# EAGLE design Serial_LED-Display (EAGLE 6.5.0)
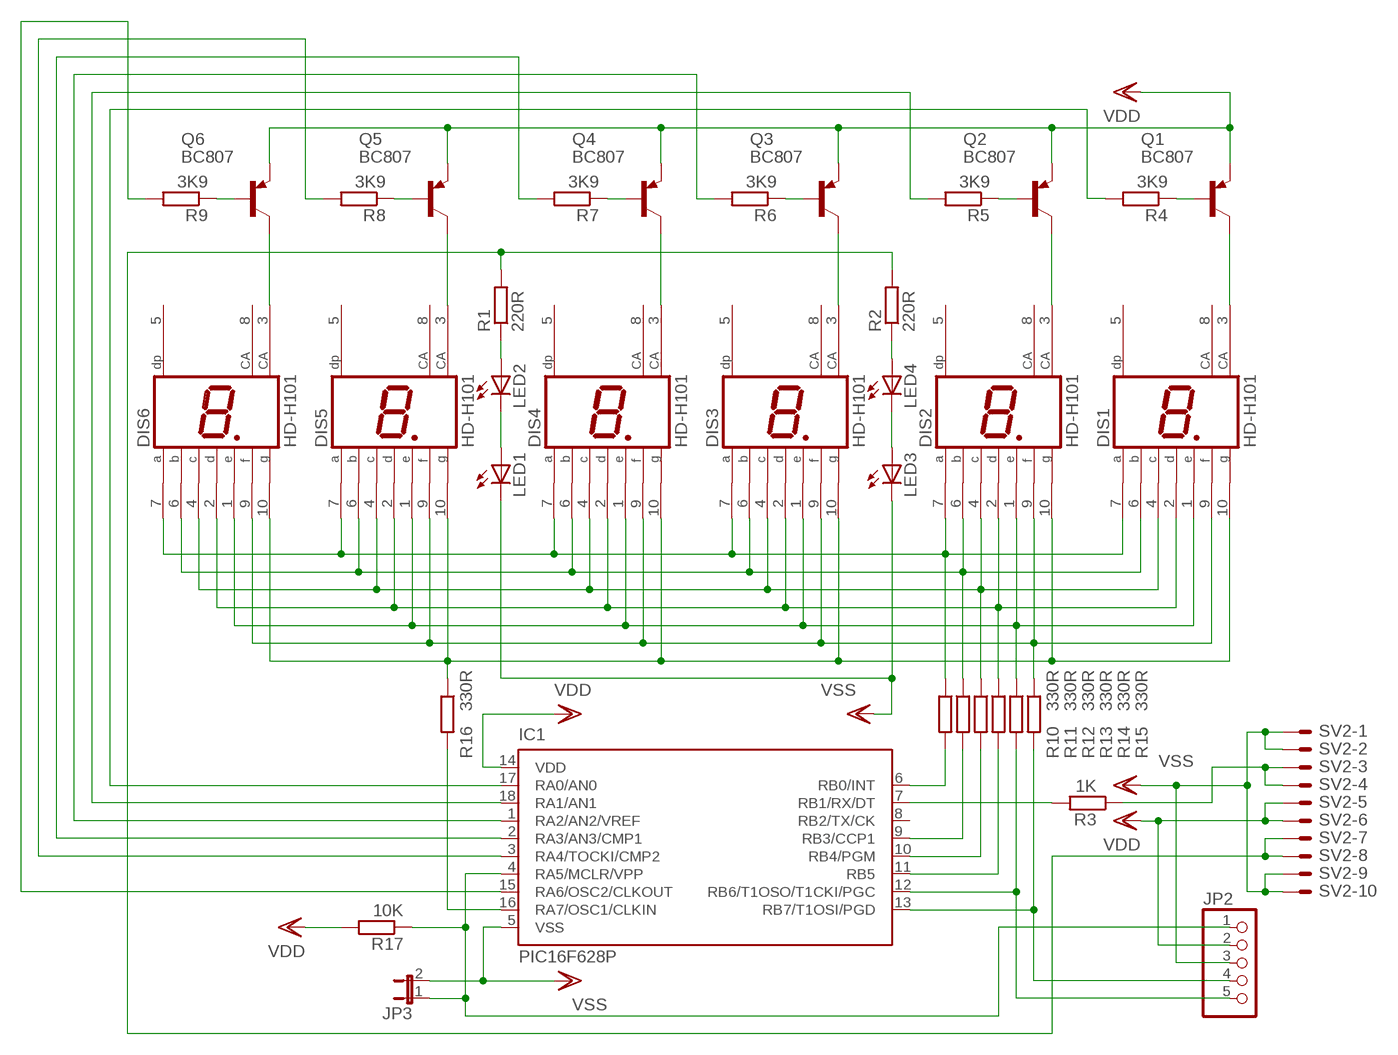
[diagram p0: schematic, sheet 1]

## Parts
DIS1  HD-H101  [HDSP-M]
DIS2  HD-H101  [HDSP-M]
DIS3  HD-H101  [HDSP-M]
DIS4  HD-H101  [HDSP-M]
DIS5  HD-H101  [HDSP-M]
DIS6  HD-H101  [HDSP-M]
IC1  PIC16F628P  [DIL18]
JP2  PINHD-1X5  [1X05]
JP3  JP1E  [JP1]
LED1  LED3MM  [LED3MM]
LED2  LED3MM  [LED3MM]
LED3  LED3MM  [LED3MM]
LED4  LED3MM  [LED3MM]
Q1  BC807  BC807-25SMD  [SOT23-BEC]
Q2  BC807  BC807-25SMD  [SOT23-BEC]
Q3  BC807  BC807-25SMD  [SOT23-BEC]
Q4  BC807  BC807-25SMD  [SOT23-BEC]
Q5  BC807  BC807-25SMD  [SOT23-BEC]
Q6  BC807  BC807-25SMD  [SOT23-BEC]
R1  220R  R-EU_R1206  [R1206]
R2  220R  R-EU_R1206  [R1206]
R3  1K  R-EU_R1206  [R1206]
R4  3K9  R-EU_R1206  [R1206]
R5  3K9  R-EU_R1206  [R1206]
R6  3K9  R-EU_R1206  [R1206]
R7  3K9  R-EU_R1206  [R1206]
R8  3K9  R-EU_R1206  [R1206]
R9  3K9  R-EU_R1206  [R1206]
R10  330R  R-EU_R1206  [R1206]
R11  330R  R-EU_R1206  [R1206]
R12  330R  R-EU_R1206  [R1206]
R13  330R  R-EU_R1206  [R1206]
R14  330R  R-EU_R1206  [R1206]
R15  330R  R-EU_R1206  [R1206]
R16  330R  R-EU_R1206  [R1206]
R17  10K  R-EU_R1206  [R1206]
SV2  ML10E  [ML10]

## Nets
N$1: DIS1.7(A) DIS2.7(A) DIS3.7(A) DIS4.7(A) DIS5.7(A) DIS6.7(A) R10.1
N$2: DIS1.6(B) DIS2.6(B) DIS3.6(B) DIS4.6(B) DIS5.6(B) DIS6.6(B) R11.1
N$3: DIS1.4(C) DIS2.4(C) DIS3.4(C) DIS4.4(C) DIS5.4(C) DIS6.4(C) R12.1
N$4: DIS1.2(D) DIS2.2(D) DIS3.2(D) DIS4.2(D) DIS5.2(D) DIS6.2(D) R13.1
N$5: DIS1.1(E) DIS2.1(E) DIS3.1(E) DIS4.1(E) DIS5.1(E) DIS6.1(E) R14.1
N$6: DIS1.9(F) DIS2.9(F) DIS3.9(F) DIS4.9(F) DIS5.9(F) DIS6.9(F) R15.1
N$7: DIS1.10(G) DIS2.10(G) DIS3.10(G) DIS4.10(G) DIS5.10(G) DIS6.10(G) R16.1
N$8: IC1.4(RA5/MCLR/VPP) JP2.1 JP3.1 R17.1
N$9: LED1.A LED2.K(C)
N$10: LED3.A LED4.K(C)
N$11: LED2.A R1.1
N$12: LED4.A R2.1
N$15: DIS1.3(CA) Q1.C
N$16: DIS2.3(CA) Q2.C
N$17: DIS3.3(CA) Q3.C
N$18: IC1.7(RB1/RX/DT) R3.2
N$19: DIS4.3(CA) Q4.C
N$20: DIS5.3(CA) Q5.C
N$21: DIS6.3(CA) Q6.C
N$22: Q6.B R9.1
N$23: Q5.B R8.1
N$24: Q4.B R7.1
N$25: Q3.B R6.1
N$26: Q2.B R5.1
N$27: Q1.B R4.1
N$28: IC1.17(RA0/AN0) R4.2
N$29: IC1.18(RA1/AN1) R5.2
N$30: IC1.1(RA2/AN2/VREF) R6.2
N$31: IC1.2(RA3/AN3/CMP1) R7.2
N$32: IC1.3(RA4/TOCKI/CMP2) R8.2
N$33: IC1.15(RA6/OSC2/CLKOUT) R9.2
N$34: IC1.9(RB3/CCP1) R11.2
N$35: IC1.6(RB0/INT) R10.2
N$36: IC1.10(RB4/PGM) R12.2
N$37: IC1.11(RB5) R13.2
N$38: IC1.12(RB6/T1OSO/T1CKI/PGC) JP2.5 R14.2
N$39: IC1.13(RB7/T1OSI/PGD) JP2.4 R15.2
N$40: IC1.16(RA7/OSC1/CLKIN) R16.2
N$45: R3.1 SV2.3 SV2.4
N$47: R1.2 R2.2 SV2.7 SV2.8
VDD: IC1.14(VDD) JP2.2 Q1.E Q2.E Q3.E Q4.E Q5.E Q6.E R17.2 SV2.5 SV2.6
VSS: IC1.5(VSS) JP2.3 JP3.2 LED1.K(C) LED3.K(C) SV2.1 SV2.2 SV2.9 SV2.10
Unconnected: DIS1.5(DP) DIS1.8(CA) DIS2.5(DP) DIS2.8(CA) DIS3.5(DP) DIS3.8(CA) DIS4.5(DP) DIS4.8(CA) DIS5.5(DP) DIS5.8(CA) DIS6.5(DP) DIS6.8(CA) IC1.8(RB2/TX/CK)

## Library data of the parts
DIS1-DIS6 = display-hp:HD-H101: LED DISPLAY 1-character 7 segment, decimal point right; OC_FARNELL: unknown; OC_NEWARK: unknown
IC1 = microchip-6:PIC16F62*: FLASH-Based 8-Bit CMOS Microcontroller Source: http://ww1.microchip.com/downloads/en/DeviceDoc/40300C.pdf
JP2 = pinhead:PINHD-1X5: PIN HEADER
JP3 = jumper:JP1E: JUMPER
LED1-LED4 = led:LED: LED
Q1-Q6 = transistor-pnp:BC807*: PNP Transistror
R1-R17 = rcl:R-EU_: RESISTOR, European symbol
SV2 = con-ml:ML10E: HARTING; OC_FARNELL: unknown; OC_NEWARK: unknown

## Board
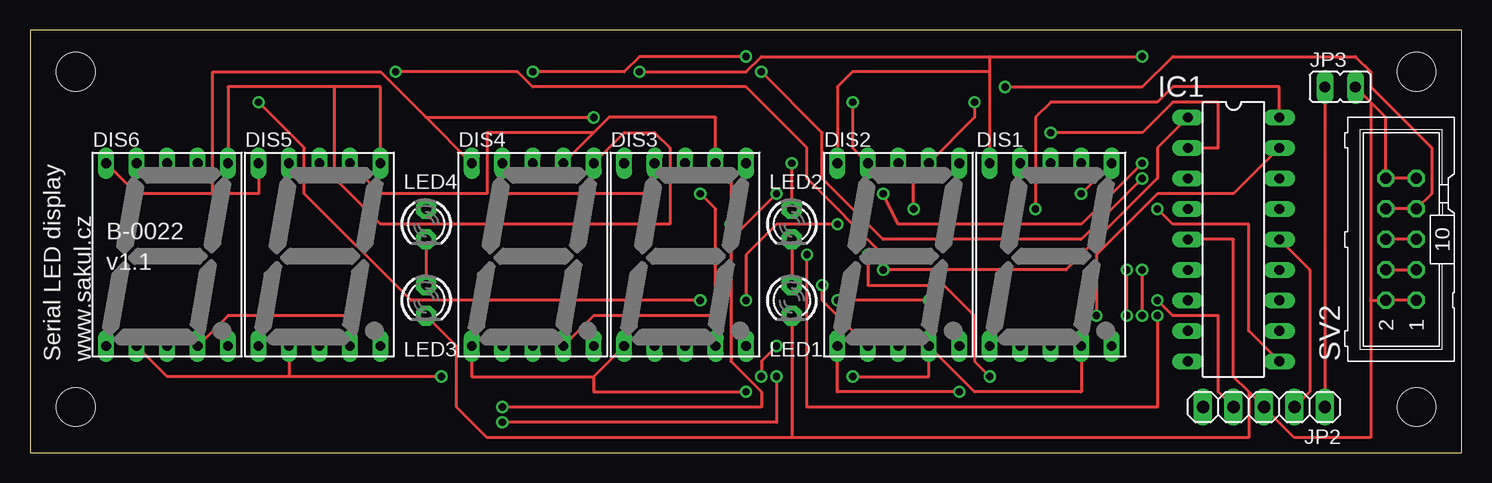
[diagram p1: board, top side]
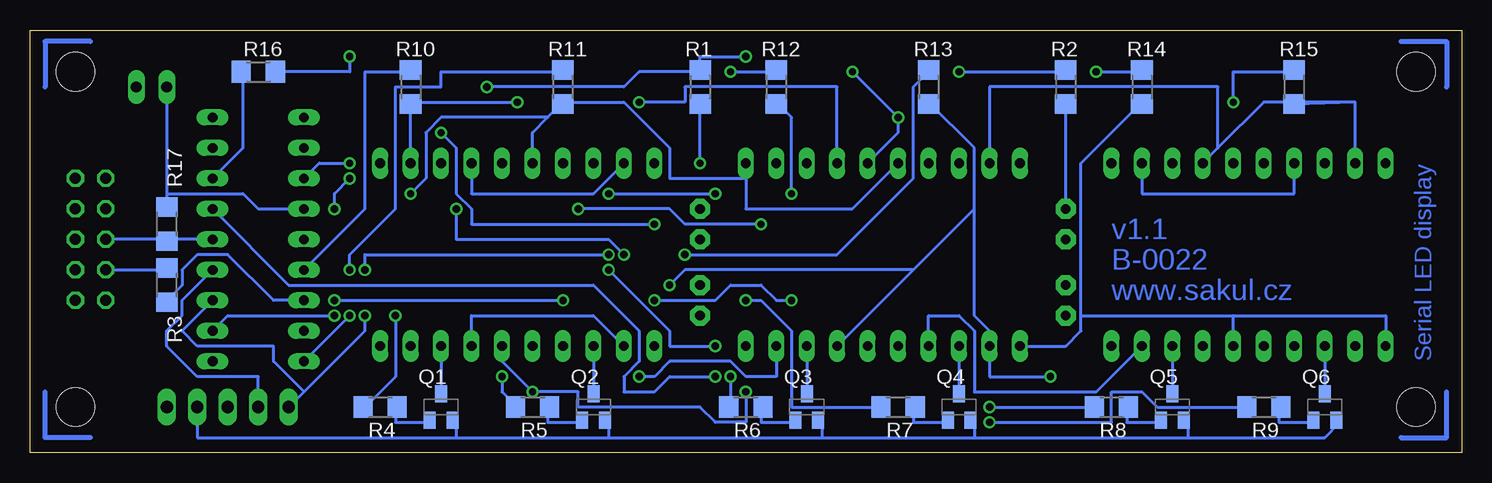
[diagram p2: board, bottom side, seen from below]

Size 119.36 x 35.23 mm. Coordinates in mm from the lower left corner, seen from the top.
Outline: 0,0 119.36,0 119.36,35.23 0,35.23 0,0
Copper layers (1*16): Top 0.035mm / dielectric 1.5mm / Bottom 0.035mm
Design rules "default": minimum track width 10mil, minimum drill 24mil, track to track 8mil, track to pad 8mil, pad to pad 8mil, via to via 8mil, smd to smd 8mil, copper to edge 40mil, drill to drill 8mil, minimum pad ring 10mil, minimum via ring 8mil, stop-mask expansion 4mil, vias tented up to drill 0mil, thermal gap 10mil
Holes 3.2 mm at 3.81,31.75 3.81,3.81 115.57,31.75 115.57,3.81

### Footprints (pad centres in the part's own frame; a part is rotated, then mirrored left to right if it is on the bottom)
HDSP-M = drill 0.813 long: 1 -5.08,-7.62; 2 -2.54,-7.62; 3 0,-7.62; 4 2.54,-7.62; 5 5.08,-7.62; 6 5.08,7.62; 7 2.54,7.62; 8 0,7.62; 9 -2.54,7.62; 10 -5.08,7.62
DIL18 = drill 0.813 long: 1 -10.16,-3.81; 2 -7.62,-3.81; 3 -5.08,-3.81; 4 -2.54,-3.81; 5 0,-3.81; 6 2.54,-3.81; 7 5.08,-3.81; 8 7.62,-3.81; 9 10.16,-3.81; 10 10.16,3.81; 11 7.62,3.81; 12 5.08,3.81; 13 2.54,3.81; 14 0,3.81; 15 -2.54,3.81; 16 -5.08,3.81; 17 -7.62,3.81; 18 -10.16,3.81
1X05 = drill 1.016 long: 1 -5.08,0; 2 -2.54,0; 3 0,0; 4 2.54,0; 5 5.08,0
JP1 = drill 0.914 long: 1 0,-1.27; 2 0,1.27
LED3MM = drill 0.813 pad 1.676 octagon: A -1.27,0; K 1.27,0
SOT23-BEC = smd 1 x 1.4: B -0.95,-1.1; C 0,1.1; E 0.95,-1.1
R1206 = smd 1.6 x 1.803: 1 -1.422,0; 2 1.422,0
ML10 = drill 0.914 octagon: 1 -5.08,-1.27; 2 -5.08,1.27; 3 -2.54,-1.27; 4 -2.54,1.27; 5 0,-1.27; 6 0,1.27; 7 2.54,-1.27; 8 2.54,1.27; 9 5.08,-1.27; 10 5.08,1.27

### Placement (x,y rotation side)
DIS1  85.09,16.51 0 top
DIS2  72.39,16.51 0 top
DIS3  54.61,16.51 0 top
DIS4  41.91,16.51 0 top
DIS5  24.13,16.51 0 top
DIS6  11.43,16.51 0 top
IC1  100.33,17.78 270 top
JP2  102.87,3.81 180 top
JP3  109.22,30.48 270 top
LED1  63.5,12.7 270 top
LED2  63.5,19.05 270 top
LED3  33.02,12.7 270 top
LED4  33.02,19.05 270 top
Q1  85.09,3.81 0 bottom
Q2  72.39,3.81 0 bottom
Q3  54.61,3.81 0 bottom
Q4  41.91,3.81 0 bottom
Q5  24.13,3.81 0 bottom
Q6  11.43,3.81 0 bottom
R1  63.5,30.48 90 bottom
R2  33.02,30.48 90 bottom
R3  107.95,13.97 270 bottom
R4  90.17,3.81 180 bottom
R5  77.47,3.81 180 bottom
R6  59.69,3.81 180 bottom
R7  46.99,3.81 180 bottom
R8  29.21,3.81 180 bottom
R9  16.51,3.81 180 bottom
R10  87.63,30.48 90 bottom
R11  74.93,30.48 90 bottom
R12  57.15,30.48 90 bottom
R13  44.45,30.48 90 bottom
R14  26.67,30.48 90 bottom
R15  13.97,30.48 90 bottom
R16  100.33,31.75 180 bottom
R17  107.95,19.05 270 bottom
SV2  114.3,17.78 90 top

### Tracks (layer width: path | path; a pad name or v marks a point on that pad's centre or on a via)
N$1  (via drill 0.61)
  Top 0.254: v78.74,29.21 78.74,27.94 DIS2.7 73.66,22.86 v73.66,20.32 | 46.99,26.67 48.26,27.94 57.15,27.94 DIS3.7 58.42,22.86 v58.42,19.05 | 46.99,26.67 DIS4.7 | DIS5.7 29.21,21.59 38.1,21.59 38.1,26.67 46.99,26.67
  Bottom 0.254: DIS1.7 R10.1 87.63,29.21 v78.74,29.21 | DIS6.7 13.97,21.59 26.67,21.59 DIS5.7 | v73.66,20.32 66.04,20.32 64.77,19.05 v58.42,19.05
N$2  (via drill 0.61)
  Top 0.254: DIS6.6 16.51,30.48 25.4,30.48 | 25.4,30.48 29.21,30.48 DIS5.6 | v87.63,21.59 DIS1.6 | 25.4,30.48 25.4,22.86 29.21,19.05 53.34,19.05 53.34,25.4 52.07,26.67 49.53,26.67 DIS4.6
  Bottom 0.254: DIS4.6 50.8,20.32 59.69,20.32 59.69,22.86 | 76.2,27.94 77.47,26.67 DIS2.6 | 76.2,27.94 74.93,29.21 | v87.63,21.59 86.36,22.86 86.36,26.67 85.09,27.94 76.2,27.94 | 59.69,22.86 66.04,22.86 66.04,25.4 69.85,29.21 74.93,29.21 | 59.69,22.86 DIS3.6 | 74.93,29.21 R11.1
N$3  (via drill 0.61)
  Top 0.254: DIS1.4 87.63,5.08 78.74,5.08 DIS2.4 74.93,6.35 v68.58,6.35 | DIS6.4 16.51,11.43 26.67,11.43 DIS5.4 | v55.88,21.59 57.15,20.32 57.15,11.43 | DIS3.4 57.15,11.43 | DIS4.4 46.99,11.43 57.15,11.43
  Bottom 0.254: v55.88,21.59 55.88,27.94 57.15,29.21 R12.1 | DIS5.4 30.48,5.08 40.64,5.08 40.64,10.16 41.91,11.43 44.45,11.43 DIS4.4 | v68.58,6.35 67.31,6.35 66.04,7.62 60.96,7.62 59.69,6.35 57.15,6.35 DIS3.4
N$4  (via drill 0.61)
  Top 0.254: DIS6.2 11.43,6.35 21.59,6.35 | DIS5.2 21.59,6.35 | v34.29,6.35 21.59,6.35 | DIS2.2 66.04,12.7 v66.04,13.97
  Bottom 0.254: DIS2.2 72.39,11.43 82.55,11.43 DIS1.2 | 40.64,20.32 40.64,11.43 39.37,10.16 DIS4.2 39.37,6.35 v34.29,6.35 | 40.64,20.32 40.64,25.4 44.45,29.21 R13.1 | 40.64,20.32 45.72,15.24 | 45.72,15.24 DIS3.2 | v66.04,13.97 64.77,15.24 45.72,15.24
N$5  (via drill 0.61)
  Top 0.254: DIS2.1 67.31,5.08 v77.47,5.08 | 46.99,6.35 DIS3.1 | 46.99,6.35 36.83,6.35 DIS4.1 | v59.69,5.08 46.99,5.08 46.99,6.35
  Bottom 0.254: DIS1.1 80.01,7.62 v77.47,5.08 73.66,5.08 73.66,3.81 63.5,3.81 62.23,2.54 59.69,2.54 v59.69,5.08 | DIS6.1 6.35,11.43 19.05,11.43 | DIS5.1 19.05,11.43 | 31.75,11.43 31.75,10.16 33.02,8.89 DIS4.1 | 31.75,11.43 31.75,24.13 26.67,29.21 R14.1 | 31.75,11.43 19.05,11.43
N$6  (via drill 0.61)
  Top 0.254: DIS4.9 39.37,21.59 52.07,21.59 DIS3.9 | DIS2.9 68.58,25.4 v68.58,29.21
  Bottom 0.254: DIS2.9 72.39,21.59 82.55,21.59 DIS1.9 | DIS6.9 8.89,29.21 | 20.32,25.4 16.51,29.21 8.89,29.21 | 20.32,25.4 DIS5.9 | 8.89,29.21 R15.1 | DIS4.9 39.37,30.48 20.32,30.48 20.32,25.4 | v68.58,29.21 64.77,29.21 64.77,30.48 52.07,30.48 DIS3.9
N$7  (via drill 0.61)
  Top 0.254: 80.01,33.02 v92.71,33.02 | DIS1.10 80.01,31.75 | 80.01,31.75 80.01,33.02 | DIS2.10 67.31,30.48 68.58,31.75 80.01,31.75 | DIS6.10 8.89,21.59 15.24,21.59 | 15.24,21.59 19.05,21.59 DIS5.10 | 33.02,27.94 29.21,31.75 15.24,31.75 15.24,21.59 | 33.02,27.94 DIS4.10 | 33.02,27.94 v46.99,27.94 | 80.01,33.02 60.96,33.02 59.69,31.75 v50.8,31.75
  Bottom 0.254: v92.71,33.02 92.71,31.75 R16.1 99.06,31.75 | DIS3.10 46.99,26.67 v46.99,27.94 v50.8,31.75
N$8
  Top 0.254: JP3.1 JP2.1
  Bottom 0.254: JP3.1 107.95,21.59 | 107.95,21.59 R17.1 107.95,20.32 | IC1.4 100.33,20.32 101.6,21.59 107.95,21.59
N$9
  Top 0.254: LED2.K LED1.A
N$10
  Top 0.254: LED4.K LED3.A
N$11  (via drill 0.61)
  Top 0.254: LED2.A v63.5,24.13
  Bottom 0.254: v63.5,24.13 R1.1 63.5,29.21
N$12
  Bottom 0.254: LED4.A R2.1 33.02,29.21
N$15
  Bottom 0.254: DIS1.3 Q1.C
N$16
  Bottom 0.254: DIS2.3 Q2.C
N$17
  Bottom 0.254: DIS3.3 Q3.C
N$18
  Bottom 0.254: IC1.7 99.06,12.7 102.87,16.51 105.41,16.51 106.68,15.24 106.68,13.97 107.95,12.7 R3.2
N$19
  Bottom 0.254: DIS4.3 Q4.C
N$20
  Bottom 0.254: DIS5.3 Q5.C
N$21
  Bottom 0.254: DIS6.3 Q6.C
N$22
  Bottom 0.254: Q6.B 12.7,2.54 15.24,2.54 15.24,3.81 R9.1
N$23
  Bottom 0.254: Q5.B 25.4,2.54 27.94,2.54 27.94,3.81 R8.1
N$24
  Bottom 0.254: Q4.B 43.18,2.54 45.72,2.54 45.72,3.81 R7.1
N$25
  Bottom 0.254: Q3.B 55.88,2.54 58.42,2.54 58.42,3.81 R6.1
N$26
  Bottom 0.254: Q2.B 73.66,2.54 76.2,2.54 76.2,3.81 R5.1
N$27
  Bottom 0.254: Q1.B 86.36,2.54 88.9,2.54 88.9,3.81 R4.1
N$28  (via drill 0.61)
  Top 0.254: v88.9,11.43 88.9,16.51 93.98,21.59 100.33,21.59 IC1.17
  Bottom 0.254: v88.9,11.43 88.9,6.35 91.44,3.81 R4.2
N$29  (via drill 0.61)
  Top 0.254: v80.01,6.35 78.74,7.62 78.74,11.43 76.2,13.97 69.85,13.97 v69.85,16.51 | v83.82,20.32 83.82,27.94 85.09,29.21 93.98,29.21 95.25,30.48 104.14,30.48 IC1.18
  Bottom 0.254: v80.01,6.35 80.01,5.08 78.74,3.81 R5.2 | v69.85,16.51 71.12,17.78 83.82,17.78 v83.82,20.32
N$30  (via drill 0.61)
  Top 0.254: v60.96,6.35 60.96,7.62 v62.23,8.89 | v71.12,15.24 86.36,15.24 93.98,22.86 93.98,25.4 IC1.1
  Bottom 0.254: v60.96,6.35 60.96,3.81 R6.2 | v62.23,8.89 66.04,8.89 66.04,10.16 v71.12,15.24
N$31  (via drill 0.61)
  Top 0.254: v59.69,12.7 59.69,16.51 62.23,19.05 v67.31,19.05 | v85.09,26.67 92.71,26.67 95.25,29.21 99.06,29.21 99.06,25.4 IC1.2
  Bottom 0.254: v59.69,12.7 58.42,12.7 55.88,10.16 55.88,3.81 R7.2 48.26,3.81 | v67.31,19.05 82.55,19.05 82.55,20.32 83.82,21.59 83.82,25.4 v85.09,26.67
N$32  (via drill 0.61)
  Top 0.254: v39.37,3.81 60.96,3.81 60.96,5.08 58.42,7.62 58.42,17.78 v62.23,21.59 | v71.12,21.59 72.39,19.05 87.63,19.05 v92.71,24.13
  Bottom 0.254: v39.37,3.81 R8.2 30.48,3.81 | v71.12,21.59 v62.23,21.59 | v92.71,24.13 95.25,24.13 IC1.3
N$33  (via drill 0.61)
  Top 0.254: v39.37,2.54 62.23,2.54 v62.23,6.35
  Bottom 0.254: v39.37,2.54 29.21,2.54 29.21,5.08 26.67,5.08 25.4,3.81 R9.2 17.78,3.81 | v62.23,6.35 66.04,6.35 67.31,5.08 69.85,5.08 69.85,6.35 68.58,7.62 68.58,10.16 72.39,13.97 97.79,13.97 IC1.15
N$34  (via drill 0.61)
  Top 0.254: v92.71,11.43 v92.71,15.24
  Bottom 0.254: v92.71,15.24 92.71,16.51 88.9,20.32 88.9,30.48 85.09,30.48 85.09,31.75 74.93,31.75 R11.2 | IC1.9 v92.71,11.43
N$35
  Bottom 0.254: IC1.6 91.44,20.32 91.44,31.75 87.63,31.75 R10.2
N$36  (via drill 0.61)
  Top 0.254: v60.96,31.75 66.04,26.67 66.04,22.86 71.12,17.78 87.63,17.78 v92.71,22.86 | v93.98,20.32 95.25,19.05 101.6,19.05 101.6,10.16 IC1.10
  Bottom 0.254: v60.96,31.75 57.15,31.75 R12.2 | v92.71,22.86 93.98,21.59 v93.98,20.32
N$37  (via drill 0.61)
  Top 0.254: v64.77,16.51 64.77,3.81 93.98,3.81 v93.98,11.43
  Bottom 0.254: v64.77,16.51 52.07,16.51 45.72,22.86 45.72,30.48 44.45,31.75 R13.2 | v93.98,11.43 102.87,11.43 IC1.11
N$38  (via drill 0.61)
  Top 0.254: v30.48,31.75 40.64,31.75 41.91,30.48 59.69,30.48 64.77,25.4 64.77,22.86 v71.12,16.51 | v91.44,11.43 v91.44,15.24
  Bottom 0.254: v30.48,31.75 26.67,31.75 R14.2 | v71.12,16.51 91.44,16.51 v91.44,15.24 | v91.44,11.43 91.44,10.16 96.52,5.08 | JP2.5 96.52,5.08 | IC1.12 106.68,10.16 105.41,8.89 99.06,8.89 99.06,7.62 96.52,5.08
N$39  (via drill 0.61)
  Top 0.254: v19.05,29.21 22.86,25.4 22.86,21.59 31.75,12.7 v55.88,12.7 | v74.93,12.7 v67.31,12.7 | v93.98,12.7 95.25,11.43 99.06,11.43 99.06,5.08 JP2.4
  Bottom 0.254: v19.05,29.21 19.05,31.75 13.97,31.75 R15.2 | v55.88,12.7 57.15,12.7 58.42,13.97 60.96,13.97 62.23,12.7 v67.31,12.7 | v93.98,12.7 v74.93,12.7 | IC1.13 106.68,12.7 106.68,11.43 107.95,10.16 107.95,8.89 105.41,6.35 100.33,6.35 JP2.4
N$40
  Bottom 0.254: IC1.16 101.6,25.4 101.6,31.75 R16.2
N$41
  Bottom 0.406: 114.3,34.29 118.11,34.29 118.11,30.48
N$42
  Bottom 0.406: 114.3,1.27 118.11,1.27 118.11,5.08
N$43
  Bottom 0.406: 5.08,34.29 1.27,34.29 1.27,30.48
N$44
  Bottom 0.406: 5.08,1.27 1.27,1.27 1.27,5.08
N$45
  Top 0.254: SV2.4 SV2.3
  Bottom 0.254: SV2.4 107.95,15.24 R3.1
N$47  (via drill 0.61)
  Top 0.254: SV2.8 SV2.7 116.84,21.59 116.84,25.4 111.76,30.48 111.76,31.75 110.49,33.02 95.25,33.02 92.71,30.48 v81.28,30.48 | v41.91,31.75 49.53,31.75 50.8,33.02 v59.69,33.02
  Bottom 0.254: v41.91,31.75 33.02,31.75 R2.2 | v59.69,33.02 63.5,33.02 R1.2 63.5,31.75 68.58,31.75 69.85,30.48 v81.28,30.48
VDD
  Top 0.254: SV2.5 SV2.6 | JP2.2 106.68,5.08 106.68,15.24 IC1.14
  Bottom 0.254: 22.86,1.27 11.43,1.27 10.16,2.54 Q6.E | 22.86,1.27 22.86,2.54 Q5.E | 53.34,1.27 40.64,1.27 | 53.34,1.27 53.34,2.54 Q3.E | 40.64,1.27 22.86,1.27 | 40.64,1.27 40.64,2.54 Q4.E | 83.82,1.27 71.12,1.27 | 83.82,1.27 83.82,2.54 Q1.E | IC1.14 107.95,17.78 | 107.95,17.78 SV2.6 | 107.95,17.78 R17.2 | 83.82,1.27 105.41,1.27 JP2.2 | 71.12,1.27 53.34,1.27 | 71.12,1.27 71.12,2.54 Q2.E
VSS
  Top 0.254: LED3.K 35.56,8.89 35.56,3.81 38.1,1.27 63.5,1.27 | LED1.K 63.5,1.27 | IC1.5 100.33,17.78 100.33,6.35 101.6,5.08 | 101.6,5.08 JP2.3 105.41,1.27 111.76,1.27 111.76,12.7 | SV2.1 SV2.2 111.76,12.7 | SV2.9 SV2.10 113.03,27.94 111.76,29.21 | 111.76,29.21 JP3.2 | 111.76,29.21 111.76,12.7 | 63.5,1.27 101.6,1.27 101.6,5.08

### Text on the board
Bottom: v1.1 | B-0022 | www.sakul.cz | Serial LED display
tPlace: B-0022 | v1.1 | Serial LED display | www.sakul.cz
